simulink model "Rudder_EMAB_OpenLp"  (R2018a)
settings: Solver=ode45  StartTime=0.0  StopTime=1  RelTol=1e-3  EnableMultiTasking=on
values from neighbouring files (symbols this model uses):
  Be = 25    [init.m]
  Ja = 2.0e-4    (= 0.0002)    [init.m]
  Je = 2.2    [init.m]
  Jm = 5.0e-5    (= 5e-05)    [init.m]
  Kdmp = 0.001    [init.m]
  Keff = 0.85    [init.m]
  Kgs = 400.0    (= 400)    [init.m]
  Ki = 5.0    (= 5)    [init.m]
  Kl = 12/Kli    (= 1800000)    [init.m]
  Kmfr = 0.03    [init.m]
  Kp = 140    [init.m]
  Krfb = 0.0005    [init.m]
  Kt = 12/Kti    (= 1674418.60465)    [init.m]
  Kv = 260    [init.m]
  Ngear = 10.2    [init.m]
  Nscrew = 0.0026    [init.m]
  R = 0.287    [init.m]    (also in lqr_des.m = diag(R))
  Wmb = 1500    [init.m]

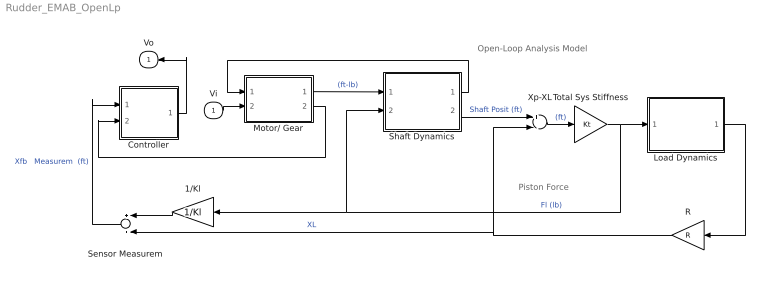
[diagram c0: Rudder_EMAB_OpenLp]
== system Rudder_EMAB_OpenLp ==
  note: Piston Force
  note: Open-Loop Analysis Model
  Vi : Inport
  1/Kl : Gain  Gain=1/Kl
  Controller : Subsystem
  Load Dynamics : Subsystem
  Motor/ Gear : Subsystem
  R : Gain  Gain=R
  Sensor Measurem : Sum
  Shaft Dynamics : Subsystem
  Total Sys Stiffness : Gain  Gain=Kt
  Xp-XL : Sum  Inputs=+-
  Vo : Outport
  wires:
  Shaft Dynamics/2(Xp) -> Xp-XL/1  "Shaft Posit (ft)"
  Xp-XL/1 -> Total Sys Stiffness/1  "(ft)"
  Total Sys Stiffness/1 -> Load Dynamics/1(FL), 1/Kl/1, Shaft Dynamics/2(FL)  "Fl (lb)"
  1/Kl/1 -> Sensor Measurem/1
  Motor/ Gear/1(Tm) -> Shaft Dynamics/1(Tq-mot)  "(ft-lb)"
  Load Dynamics/1(Delta (rad)) -> R/1
  Sensor Measurem/1 -> Controller/1(Xp-fb)  "Xfb   Measurem  (ft)"
  Shaft Dynamics/1(Xp-dot) -> Motor/ Gear/1(Xp-dot)
  R/1 -> Sensor Measurem/2, Xp-XL/2  "XL"
  Motor/ Gear/2(mr) -> Controller/2(rotor)
  Vi/1 -> Motor/ Gear/2(Vin)
  Controller/1(V) -> Vo/1

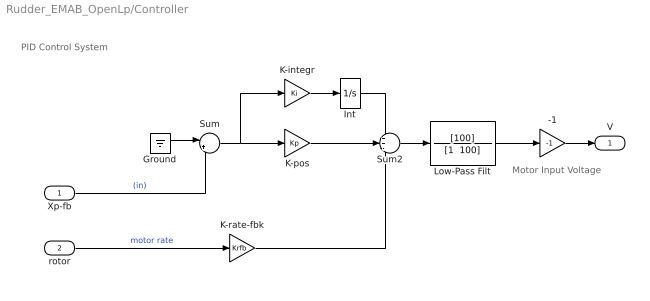
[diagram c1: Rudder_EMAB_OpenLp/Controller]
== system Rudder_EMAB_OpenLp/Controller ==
  note: PID Control System
  note: Motor Input Voltage
  Xp-fb : Inport
  rotor : Inport  Port=2
  -1 : Gain  Gain=-1
  Ground : Ground
  Int : Integrator  UpperSaturationLimit=1  LowerSaturationLimit=-1
  K-integr : Gain  Gain=Ki
  K-pos : Gain  Gain=Kp
  K-rate-fbk : Gain  Gain=Krfb
  Low-Pass Filt : TransferFcn  Numerator=[100]  Denominator="[1  100]"
  Sum : Sum  Inputs=|+-
  Sum2 : Sum  Inputs=++-
  V : Outport
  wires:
  K-rate-fbk/1 -> Sum2/3
  Int/1 -> Sum2/1
  K-integr/1 -> Int/1
  K-pos/1 -> Sum2/2
  Sum2/1 -> Low-Pass Filt/1
  rotor/1 -> K-rate-fbk/1  "motor rate"
  Sum/1 -> K-integr/1, K-pos/1
  Xp-fb/1 -> Sum/2  "(in)"
  Low-Pass Filt/1 -> -1/1
  -1/1 -> V/1
  Ground/1 -> Sum/1

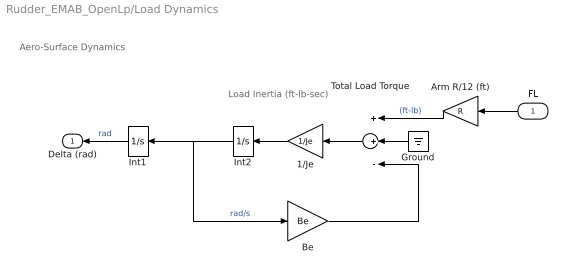
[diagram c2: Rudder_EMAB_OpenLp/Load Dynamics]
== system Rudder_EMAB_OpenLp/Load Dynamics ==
  note: Aero-Surface Dynamics
  note: Load Inertia (ft-lb-sec)
  FL : Inport
  1/Je : Gain  Gain=1/Je
  Arm R/12 (ft) : Gain  Gain=R
  Be : Gain  Gain=Be
  Ground : Ground
  Int1 : Integrator
  Int2 : Integrator
  Total Load Torque : Sum  Inputs=++-
  Delta (rad) : Outport
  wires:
  Be/1 -> Total Load Torque/3
  Total Load Torque/1 -> 1/Je/1
  Int1/1 -> Delta (rad)/1  "rad"
  Int2/1 -> Be/1, Int1/1  "rad/s"
  1/Je/1 -> Int2/1
  FL/1 -> Arm R/12 (ft)/1
  Arm R/12 (ft)/1 -> Total Load Torque/1  "(ft-lb)"
  Ground/1 -> Total Load Torque/2

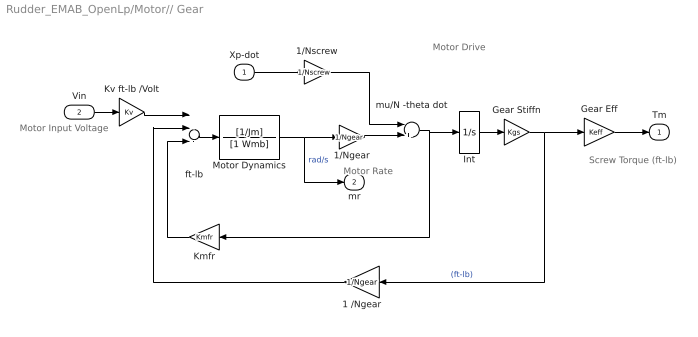
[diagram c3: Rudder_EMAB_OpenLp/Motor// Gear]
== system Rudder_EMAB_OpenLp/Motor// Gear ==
  note: Motor Drive
  note: Motor Input Voltage
  note: Motor Rate
  note: Screw Torque (ft-lb)
  Xp-dot : Inport
  Vin : Inport  Port=2
  1 /Ngear : Gain  Gain=1/Ngear
  1/Ngear : Gain  Gain=1/Ngear
  1/Nscrew : Gain  Gain=1/Nscrew
  Gear Eff : Gain  Gain=Keff
  Gear Stiffn : Gain  Gain=Kgs
  Int : Integrator  UpperSaturationLimit=0.4  LowerSaturationLimit=-0.4
  Kmfr : Gain  Gain=Kmfr
  Kv ft-lb /Volt : Gain  Gain=Kv
  Motor Dynamics : TransferFcn  Numerator=[1/Jm]  Denominator=[1 Wmb]
  ft-lb : Sum  Inputs=+---
  mu/N -theta dot : Sum  Inputs=-+
  Tm : Outport
  mr : Outport  Port=2
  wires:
  mu/N -theta dot/1 -> Int/1, Kmfr/1
  ft-lb/1 -> Motor Dynamics/1
  1 /Ngear/1 -> ft-lb/2
  Motor Dynamics/1 -> 1/Ngear/1, mr/1  "rad/s"
  1/Ngear/1 -> mu/N -theta dot/2
  Gear Stiffn/1 -> 1 /Ngear/1, Gear Eff/1  "(ft-lb)"
  Xp-dot/1 -> 1/Nscrew/1
  Vin/1 -> Kv ft-lb /Volt/1
  Gear Eff/1 -> Tm/1
  Kv ft-lb /Volt/1 -> ft-lb/1
  1/Nscrew/1 -> mu/N -theta dot/1
  Kmfr/1 -> ft-lb/3
  Int/1 -> Gear Stiffn/1

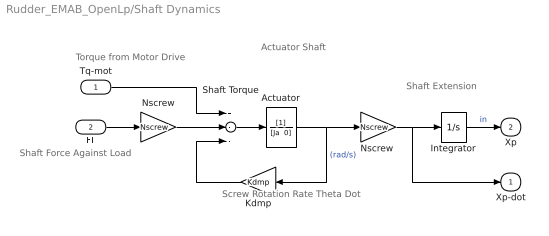
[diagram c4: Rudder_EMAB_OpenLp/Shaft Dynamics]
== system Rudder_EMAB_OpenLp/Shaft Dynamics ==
  note: Actuator Shaft
  note: Torque from Motor Drive
  note: Shaft Force Against Load
  note: Screw Rotation Rate Theta Dot
  note: Shaft Extension
  Tq-mot : Inport
  FL : Inport  Port=2
  Actuator : TransferFcn  Denominator="[Ja  0]"
  Integrator : Integrator
  Kdmp : Gain  Gain=Kdmp
  Nscrew : Gain  Gain=Nscrew
  "Nscrew " : Gain  Gain=Nscrew
  Shaft Torque : Sum  Inputs=+--
  Xp-dot : Outport
  Xp : Outport  Port=2
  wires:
  Actuator/1 -> "Nscrew "/1, Kdmp/1  "(rad/s)"
  Shaft Torque/1 -> Actuator/1
  Tq-mot/1 -> Shaft Torque/1
  Integrator/1 -> Xp/1  "in"
  FL/1 -> Nscrew/1
  Nscrew/1 -> Shaft Torque/2
  "Nscrew "/1 -> Integrator/1, Xp-dot/1
  Kdmp/1 -> Shaft Torque/3
